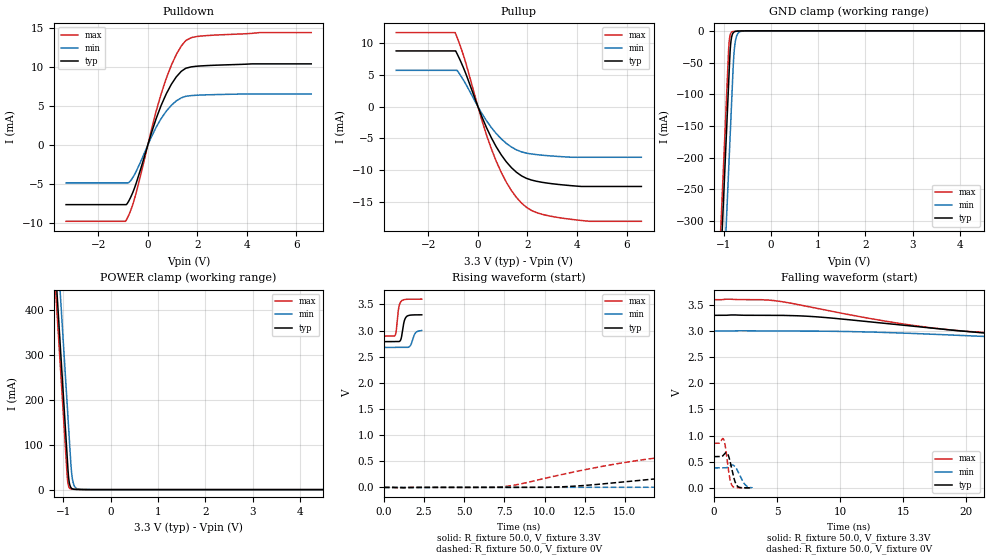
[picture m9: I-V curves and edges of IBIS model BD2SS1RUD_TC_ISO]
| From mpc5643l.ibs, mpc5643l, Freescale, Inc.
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| *** New cell (Generated with 5.14beta1 (Sep 20 2010 13:23:23))
[Model]   BD2SS1RUD_TC_ISO
Model_type I/O
Polarity   Non-Inverting
Enable   Active-Low
| CAP_THRESHOLD on pad pad is "CMOS" :
| Rising=10.0% of VDDE1   Falling=90.0% of VDDE1
| C_comp min and max val. don't necessarily correlate with the min and max pvt
| but are the smallest and greatest pad capacitance found.
| var   typ   min   max
C_comp   1.96493pF  1.84819pF  2.09390pF
Vinl = 1.05V | Dummy value overriden by next lines
Vinh = 2.34V | Dummy value overriden by next lines
Vmeas = 1.65V   | Reference voltage for timing measurements
Cref  = 25.0pF   | Timing specification test load capacitance value
Rref  = 1.0MOhm   | Timing specification test load resistance value
Vref  = 1.65V   | Timing specification test load voltage
[Model Spec]
| TIME_THRESHOLD on pin ipp_ind is "CORE" :
| Rising=40.0% of VDD   Falling=60.0% of VDD
Vinl 1.32350V 1.20950V 1.42250V
Vinh 1.90350V 1.72650V 2.05550V
| variable   typ   min   max
[Temperature Range] 25.0 150.0 -40.0
| variable   typ   min   max
[Voltage Range] 3.3V 3.0V 3.6V
| variable   typ   min   max
[POWER Clamp Reference] 3.3V 3.0V 3.6V
| variable   typ   min   max
[GND Clamp Reference] 0V 0V 0V
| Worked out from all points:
|   slope of the pulldown table from 0 to 0.495 V, typ, clamps not added: 105 ohm
|   slope of the pullup table from 0 to 0.495 V, typ, clamps not added: 110 ohm
|   GND clamp passes 1 mA (typ) near -0.75 V on its own axis
|   POWER clamp passes 1 mA (typ) near -0.78 V on its own axis
|   rising waveform, R_fixture 50.0, V_fixture 3.3V: 20-80 % time 179ps typ, 225ps min, 158ps max; typ from 2.79 V to 3.3 V
|   falling waveform, R_fixture 50.0, V_fixture 3.3V: 20-80 % time 14.5ns typ, 22.2ns min, 10.6ns max; typ from 3.3 V to 2.79 V
|   rising waveform, R_fixture 50.0, V_fixture 0V: 20-80 % time 17.6ns typ, 34.1ns min, 10.8ns max; typ from 0 V to 0.598 V
|   falling waveform, R_fixture 50.0, V_fixture 0V: 20-80 % time 363ps typ, 501ps min, 294ps max; typ from 0.598 V to 0 V
[POWER Clamp]
-3.3V     4.123A     4.24A      4.08A
-1.21V    570.2mA    687.2mA    526.7mA
-1.14V    451.2mA    568.2mA    407.7mA
-1.07V    332.2mA    449.2mA    288.7mA
-1V       213.2mA    330.2mA    169.7mA
-920mV    77.24mA    194.2mA    33.73mA
-890mV    29.56mA    143.2mA    8.381mA
-850mV    6.786mA    75.21mA    1.909mA
-820mV    2.53mA     33.85mA    1.021mA
-790mV    1.151mA    15.13mA    740.2uA
-650mV    252.6uA    576.9uA    284uA
6.6V      0A         0A         0A
[GND Clamp]
-3.3V     -4.176A    -4.313A    -4.122A
-1.08V    -402.1mA   -539.1mA   -348.2mA
-900mV    -96.14mA   -233.1mA   -42.21mA
-880mV    -62.14mA   -199.1mA   -16.29mA
-860mV    -30.87mA   -165.1mA   -6.653mA
-840mV    -14.61mA   -131.1mA   -3.031mA
-810mV    -5.028mA   -80.13mA   -1.291mA
-780mV    -1.975mA   -36.74mA   -799.8uA
-750mV    -958.4uA   -16.44mA   -596.2uA
-700mV    -452.7uA   -4.486mA   -391.1uA
-610mV    -183.2uA   -608.3uA   -147uA
6.6V      1.761nA    514.5nA    13.26pA
| variable   typ   min   max
[Pullup Reference] 3.3V 3.0V 3.6V
| variable   typ   min   max
[Pulldown Reference] 0V 0V 0V
[Pullup]
-3.3V     8.741mA    5.69mA     11.62mA
-920mV    8.741mA    5.69mA     11.62mA
-840mV    8.28mA     5.69mA     10.85mA
-530mV    5.566mA    3.805mA    7.356mA
340mV     -3.244mA   -2.186mA   -4.38mA
740mV     -6.314mA   -4.235mA   -8.575mA
950mV     -7.623mA   -5.095mA   -10.39mA
1.35V     -9.57mA    -6.34mA    -13.16mA
1.96V     -11.26mA   -7.305mA   -15.81mA
2.57V     -11.87mA   -7.617mA   -16.88mA
3.78V     -12.41mA   -7.948mA   -17.7mA
6.6V      -12.53mA   -7.952mA   -18mA
[Pulldown]
-3.3V     -7.66mA    -4.864mA   -9.801mA
-890mV    -7.66mA    -4.864mA   -9.757mA
-740mV    -7.02mA    -4.748mA   -8.788mA
-530mV    -5.459mA   -3.757mA   -6.829mA
340mV     3.416mA    2.301mA    4.375mA
740mV     6.54mA     4.322mA    8.511mA
1.15V     8.755mA    5.665mA    11.62mA
1.55V     9.877mA    6.265mA    13.45mA
1.96V     10.12mA    6.393mA    13.93mA
2.57V     10.23mA    6.464mA    14.1mA
4.52V     10.42mA    6.554mA    14.45mA
6.6V      10.42mA    6.554mA    14.45mA
[Ramp]
dV/dt_r 358.56332mV/17.61938ns 228.8942mV/34.11605ns 511.6648mV/10.75565ns
dV/dt_f 307.81842mV/14.48841ns 194.17042mV/22.15353ns 424.6048mV/10.60414ns
R_load = 50.0
| Removed startup time: 0s 0s 0s  .
| Removed end time: 2.353ns.
[Rising Waveform]
R_fixture   = 50.0
V_fixture   = 3.3V
V_fixture_min = 3.0V
V_fixture_max = 3.6V
0s        2.787V     2.676V     2.892V
705ps     2.787V     2.676V     2.913V
770ps     2.787V     2.676V     3.009V
917ps     2.787V     2.676V     3.426V
1.072ns   2.847V     2.676V     3.56V
1.242ns   3.153V     2.676V     3.589V
1.373ns   3.255V     2.676V     3.596V
1.653ns   3.294V     2.714V     3.599V
1.98ns    3.299V     2.96V      3.6V
2.355ns   3.3V       3V         3.6V
| Removed startup time: 0s 0s 0s  .
| Removed end time: 99.7ns.
[Falling Waveform]
R_fixture   = 50.0
V_fixture   = 3.3V
V_fixture_min = 3.0V
V_fixture_max = 3.6V
0s        3.3V       3V         3.6V
4.75ns    3.3V       3V         3.582V
8.5ns     3.265V     2.997V     3.417V
13.1ns    3.156V     2.976V     3.208V
16.45ns   3.073V     2.947V     3.085V
19.95ns   2.993V     2.912V     2.996V
24.15ns   2.915V     2.867V     2.946V
32.25ns   2.839V     2.789V     2.913V
47.8ns    2.802V     2.716V     2.897V
99.8ns    2.787V     2.676V     2.892V
| Removed startup time: 0s 0s 0s  .
| Removed end time: 129.8ns.
[Rising Waveform]
R_fixture   = 50.0
V_fixture   = 0V
V_fixture_min = 0V
V_fixture_max = 0V
0s        13.19nV    306.7nV    12.29nV
7.35ns    -54.33uV   -6.616uV   11.16mV
11.55ns   17.76mV    -34.63uV   277.7mV
14.5ns    93.37mV    142.1uV    452.1mV
17.95ns   191.5mV    6.755mV    601mV
23.1ns    319.8mV    41.72mV    731.4mV
29.5ns    434.6mV    100.6mV    805.9mV
43ns      549.5mV    212.2mV    844.9mV
66.8ns    591.4mV    323.6mV    852.1mV
129.9ns   597.6mV    381.5mV    852.8mV
| Removed startup time: 0s 0s 0s  .
| Removed end time: 3.021ns.
[Falling Waveform]
R_fixture   = 50.0
V_fixture   = 0V
V_fixture_min = 0V
V_fixture_max = 0V
0s        597.6mV    381.8mV    852.8mV
774ps     636.6mV    381.8mV    921.9mV
901ps     668.7mV    381.8mV    782.8mV
1.092ns   644mV      397.6mV    429.8mV
1.282ns   493.3mV    425.7mV    140.3mV
1.46ns    300.9mV    436.2mV    33.3mV
1.673ns   110.7mV    403.6mV    5.964mV
1.88ns    26.52mV    320.8mV    1.472mV
2.448ns   708.2uV    65.49mV    178.4uV
3.023ns   84.32uV    55.1uV     155.6uV
